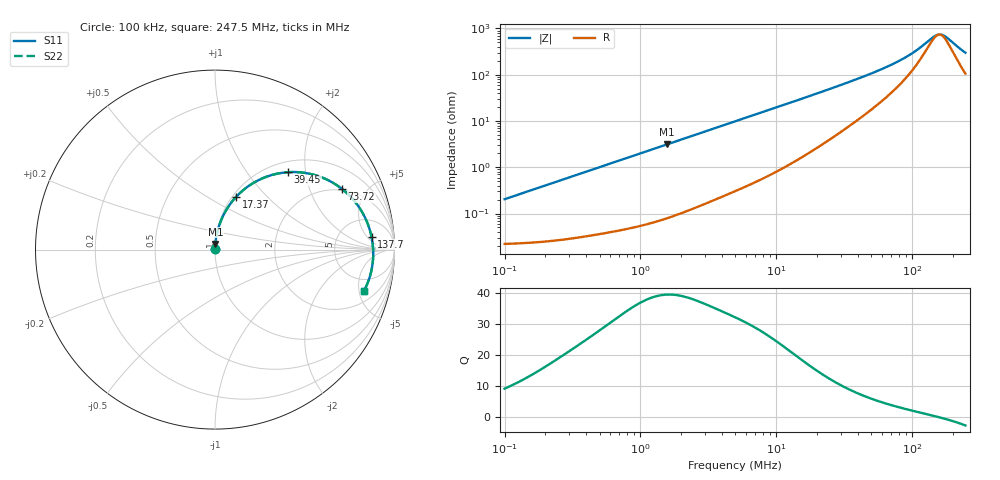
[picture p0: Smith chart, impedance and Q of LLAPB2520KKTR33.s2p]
! LLAPB2520KKTR33  S-PARAMETER MODEL  ( General Type )
! Model Generated by TAIYO YUDEN Corporation (http://www.ty-top.com)
! Version 2.0
! TAIYO YUDEN Control No. 20210629
! Copyright(c) 2015 TAIYO YUDEN CO.,LTD. All Rights Reserved.
! Product Description (link to TY-COMPAS)
! https://ds.yuden.co.jp/TYCOMPAS/or/detail?pn=LLAPB2520KKTR33M&u=M
! Products Name : Inductors
! Characteristics :
!  Inductance : 0.33 uH , SRF(min) : -Hz , DC Resistance(max) : 0.026 Ohm
!  Rated Current : Saturation :6200 mA , Temp Rise : 4300 mA (40 degC)
!  Case Size : 2.5 x 2.0 / 0.098 x 0.079 [mm/inch] , Thickness : 1 / 0.039 [mm/inch]
!  (Conditions: Temperature = 25 degC , DC Bias Current/Voltage = 0A / 0V)
! External Node Assignments :
!  1  o---GGG---o  2
! GND o---------o GND
! Frequency Range : 0.1MHz  -  247.502633MHz  [ 402 STEP ]
# MHz S RI R 50
! Freq[MHz].  S11 Real  S11 Imag  S21 Real  S21 Imag  S12 Real  S12 Imag  S22 Real  S22 Imag
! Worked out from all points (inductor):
!   401 points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, 100 kHz to 247.5 MHz, reference 50 ohm
!   read as one part in series: L = 323 nH near 104 kHz
!   highest Q = 39.5 at 1.571 MHz (marker M1), where L = 316 nH
!   self-resonance near 158.6 MHz
!   S11 on the Smith chart (normalised r, x): 100 kHz: 1.00, +0.00; 17.37 MHz: 1.04, +0.68; 39.45 MHz: 1.21, +1.61; 73.72 MHz: 1.92, +3.38; 137.7 MHz: 11, +7; 247.5 MHz: 3.12, -5.59
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0.1  0.000225 0.00203  0.9998 -0.00203  0.9998 -0.00203  0.000225 0.00203
0.37019  0.000367 0.00746  0.9996 -0.00746  0.9996 -0.00746  0.000367 0.00746
1.370406  0.00144 0.0272  0.9986 -0.0272  0.9986 -0.0272  0.00144 0.0272
1.57122  0.00176 0.0312  0.9982 -0.0312  0.9982 -0.0312  0.00176 0.0312
4.974964  0.0124 0.0962  0.9876 -0.0962  0.9876 -0.0962  0.0124 0.0962
10.24934  0.0459 0.1896  0.9541 -0.1896  0.9541 -0.1896  0.0459 0.1896
17.36851  0.1183 0.2946  0.8817 -0.2946  0.8817 -0.2946  0.1183 0.2946
18.41681  0.1309 0.3075  0.8691 -0.3075  0.8691 -0.3075  0.1309 0.3075
26.69375  0.2392 0.3854  0.7608 -0.3854  0.7608 -0.3854  0.2392 0.3854
39.45378  0.4074 0.4313  0.5926 -0.4313  0.5926 -0.4313  0.4074 0.4313
51.86374  0.5438 0.4187  0.4562 -0.4187  0.4562 -0.4187  0.5438 0.4187
68.1772  0.6737 0.3621  0.3263 -0.3621  0.3263 -0.3621  0.6737 0.3621
73.71824  0.7069 0.3385  0.2931 -0.3385  0.2931 -0.3385  0.7069 0.3385
100.767  0.8137 0.219  0.1863 -0.219  0.1863 -0.219  0.8137 0.219
115.5329  0.8455 0.1571  0.1545 -0.1571  0.1545 -0.1571  0.8455 0.1571
137.7404  0.872 0.0719  0.128 -0.0719  0.128 -0.0719  0.872 0.0719
151.8732  0.8795 0.0224  0.1205 -0.0224  0.1205 -0.0224  0.8795 0.0224
161.0397  0.8814 -0.00782  0.1186 0.00782  0.1186 0.00782  0.8814 -0.00782
167.456  0.8816 -0.0281  0.1184 0.0281  0.1184 0.0281  0.8816 -0.0281
181.0659  0.8791 -0.0691  0.1209 0.0691  0.1209 0.0691  0.8791 -0.0691
224.4709  0.852 -0.182  0.148 0.182  0.148 0.182  0.852 -0.182
247.5026  0.8292 -0.2318  0.1708 0.2318  0.1708 0.2318  0.8292 -0.2318
